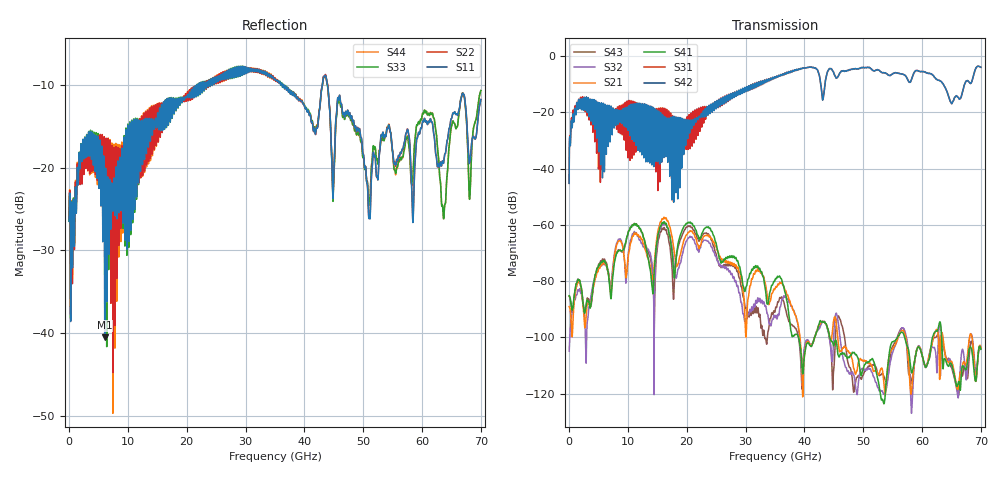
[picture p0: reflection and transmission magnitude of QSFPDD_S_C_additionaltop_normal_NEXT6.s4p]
! AWR Design Environment (8415) Thu Dec 20 13:47:57 2018
! Document = 'CHANNEL TEST'
! nPorts: 4, nXvals: 7001
# HZ S DB R 50
!Freq DBS11 AngS11 DBS12 AngS12 DBS13 AngS13 DBS14 AngS14
!	DBS21 AngS21 DBS22 AngS22 DBS23 AngS23 DBS24 AngS24
!	DBS31 AngS31 DBS32 AngS32 DBS33 AngS33 DBS34 AngS34
!	DBS41 AngS41 DBS42 AngS42 DBS43 AngS43 DBS44 AngS44
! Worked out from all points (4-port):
!   7000 points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, 10 MHz to 70 GHz, reference 50 ohm
!   strongest paths, dB at 10 MHz, 17.51 GHz, 35.01 GHz, 52.51 GHz, 70 GHz:
!     S42: -45.2, -28.8, -7.5, -5.0, -4.0
!     S31: -45.3, -23.9, -7.5, -5.0, -4.0
!     S41: -85.2, -69.8, -79.6, -114.9, -104.2
!     S21: -89.0, -64.2, -82.7, -112.9, -103.5
!     S32: -104.9, -68.0, -93.0, -117.8, -103.4
!     S43: -85.3, -75.5, -90.7, -112.7, -104.0
!   lowest |S11| = -40.5 dB at 6.06 GHz (marker M1), VSWR 1.02, Z = 49.4 + j0.738 ohm
!   |S11| at or under -10 dB: start of sweep to 21.77 GHz; 36.5 GHz to 43.04 GHz (6.538 GHz wide, 16.4 % of centre); 43.94 GHz to end of sweep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
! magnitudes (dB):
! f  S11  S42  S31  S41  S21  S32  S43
! 10 MHz  -26.5  -45.2  -45.3  -85.2  -89.0  -104.9  -85.3
! 6.06 GHz  -40.5  -22.7  -18.8  -72.8  -73.4  -73.7  -72.3
! 11.39 GHz  -16.6  -30.5  -24.8  -59.7  -62.9  -62.7  -59.6
! 14.17 GHz  -15.9  -19.0  -22.2  -83.1  -78.8  -75.0  -76.1
! 16.2 GHz  -15.3  -22.4  -20.1  -59.0  -57.4  -59.5  -61.1
! 18.26 GHz  -12.4  -22.4  -24.2  -70.7  -74.8  -78.7  -71.1
! 70 GHz  -11.8  -4.0  -4.0  -104.2  -103.5  -103.4  -104.0
